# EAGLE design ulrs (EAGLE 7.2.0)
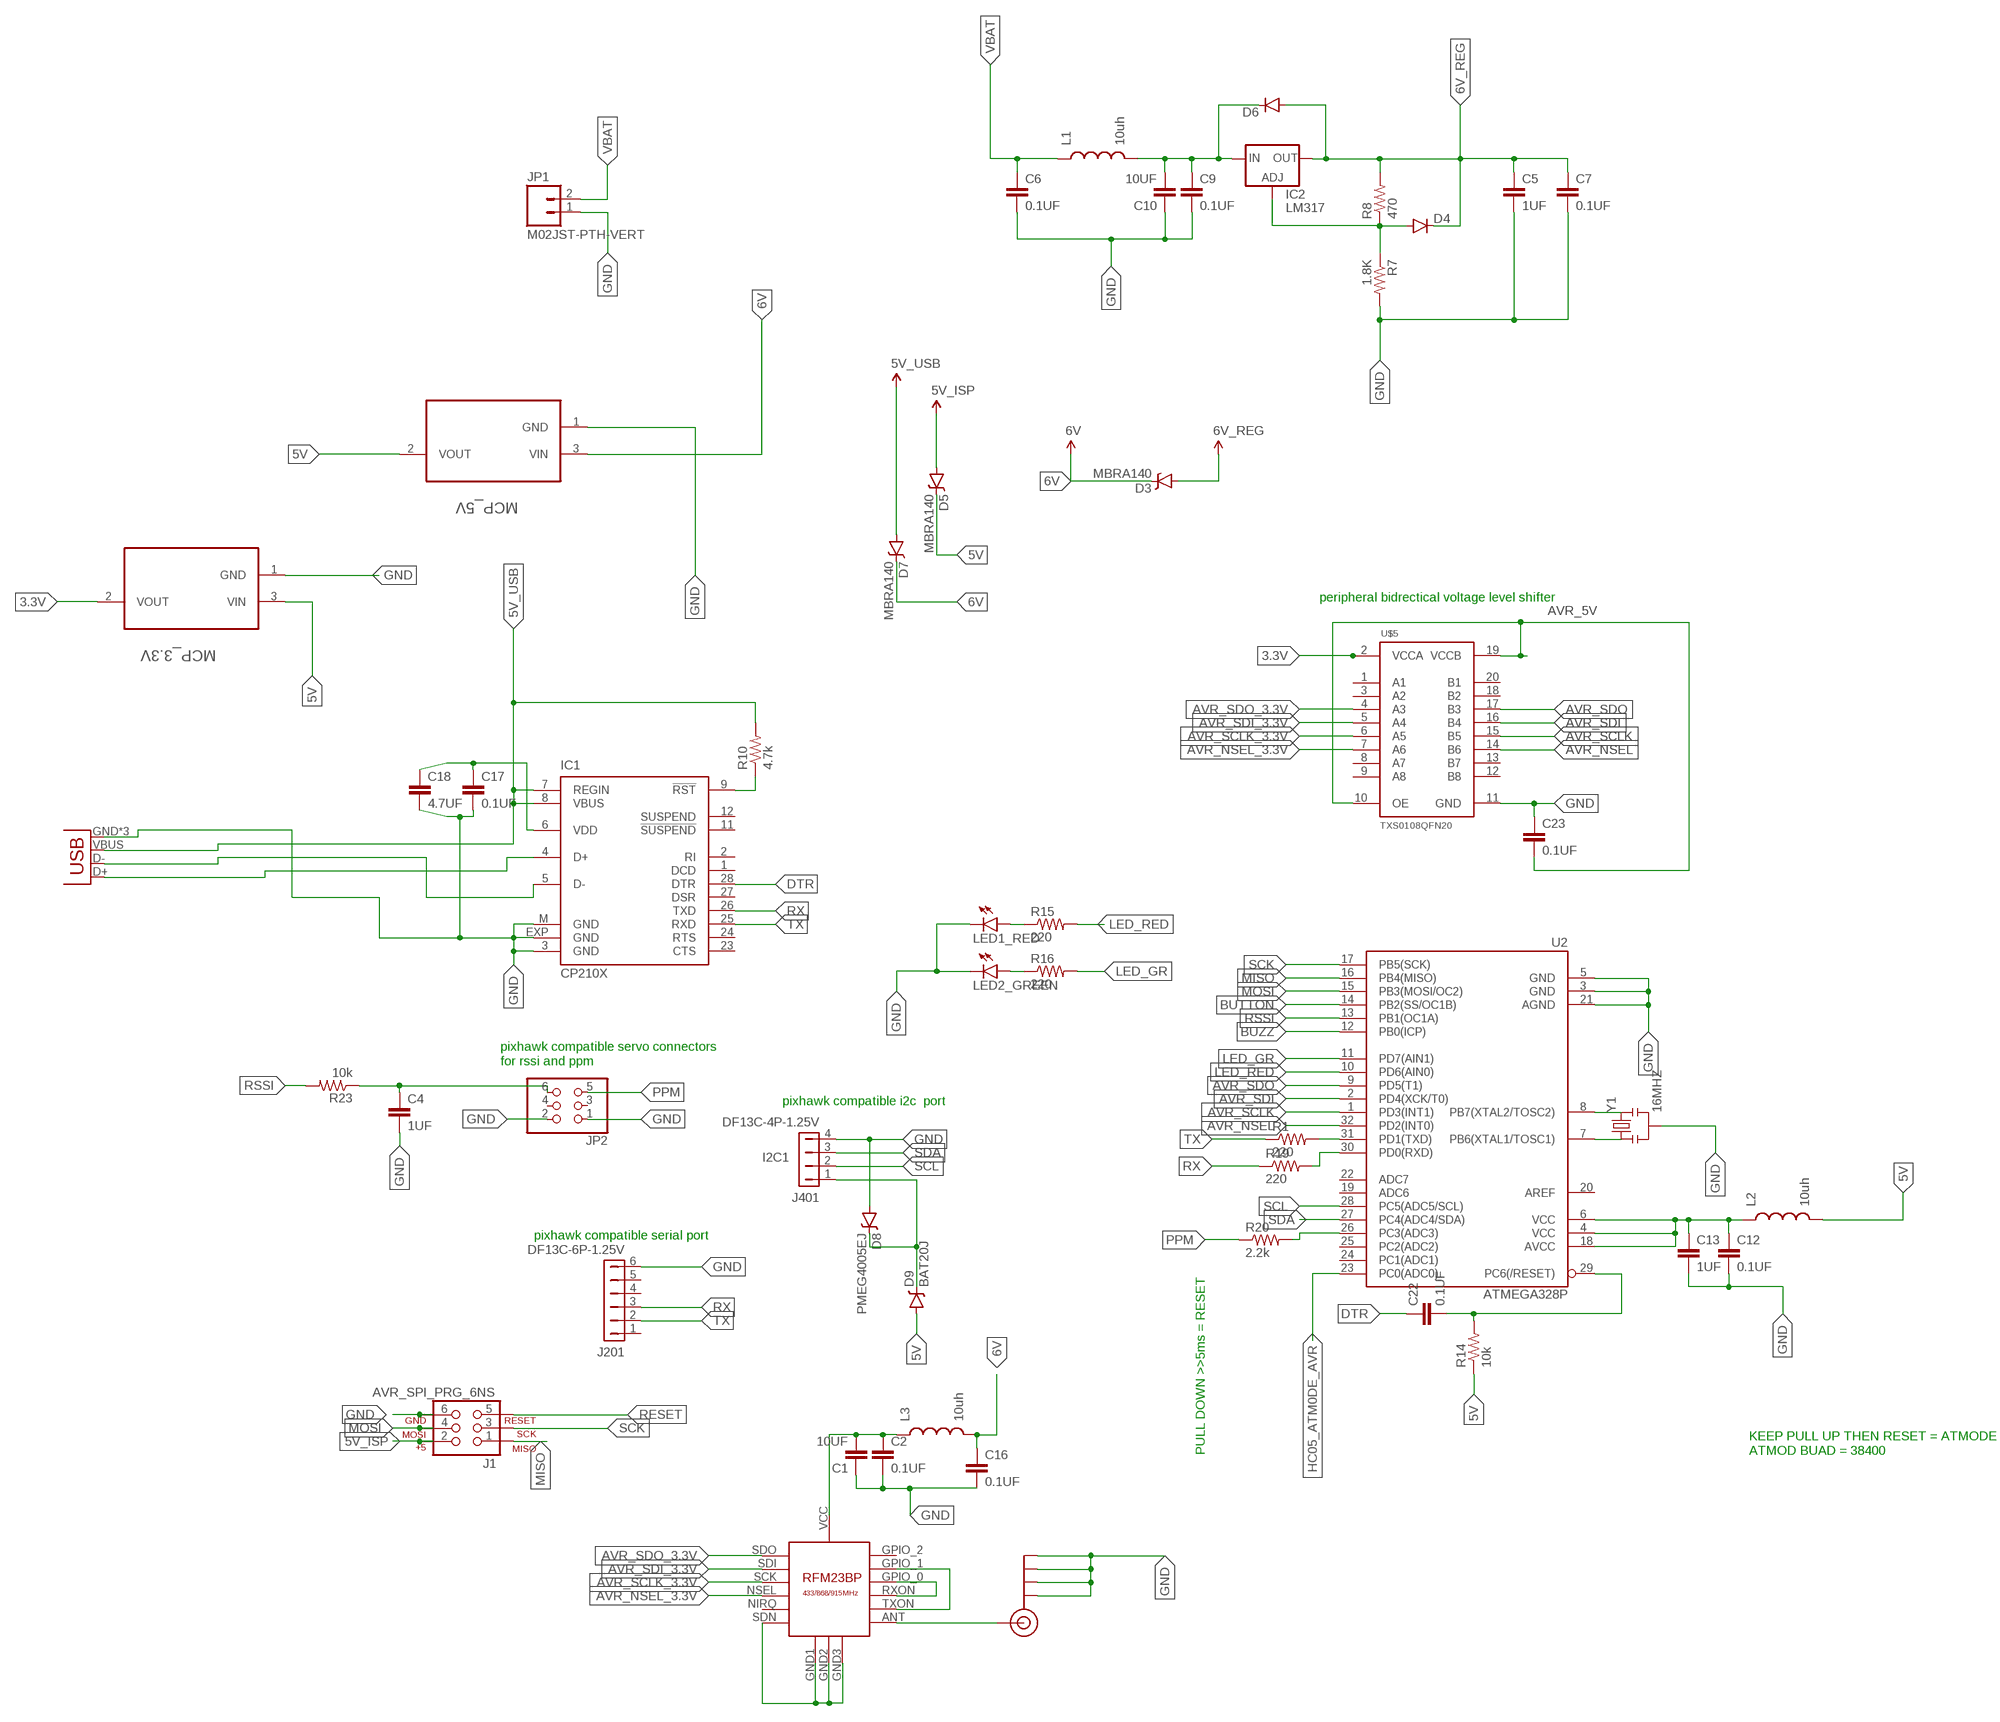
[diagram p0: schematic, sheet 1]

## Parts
C1  10UF  CAP0805  [0805]
C2  0.1UF  CAP0402-CAP  [0402-CAP]
C4  1UF  CAP0402-CAP  [0402-CAP]
C5  1UF  CAP0402-CAP  [0402-CAP]
C6  0.1UF  CAP0402-CAP  [0402-CAP]
C7  0.1UF  CAP0402-CAP  [0402-CAP]
C9  0.1UF  CAP0402-CAP  [0402-CAP]
C10  10UF  CAP1206  [1206]
C12  0.1UF  CAP0402-CAP  [0402-CAP]
C13  1UF  CAP0402-CAP  [0402-CAP]
C16  0.1UF  CAP0402-CAP  [0402-CAP]
C17  0.1UF  CAP0402-CAP  [0402-CAP]
C18  4.7UF  CAP0402-CAP  [0402-CAP]
C22  0.1UF  CAP0402-CAP  [0402-CAP]
C23  0.1UF  CAP0402-CAP  [0402-CAP]
D3  MBRA140  DIODE-SCHOTTKY-MBRA140  [SMA-DIODE]
D4  DIODESMA  [SMA-DIODE]
D5  MBRA140  DIODE-SCHOTTKY-MBRA140  [SMA-DIODE]
D6  DIODESMA  [SMA-DIODE]
D7  MBRA140  DIODE-SCHOTTKY-MBRA140  [SMA-DIODE]
D8  PMEG4005EJ  DIODE-SCHOTTKY-PMEG4005EJ  [SOD-323]
D9  BAT20J  DIODE-SCHOTTKY-BAT20J  [SOD-323]
IC1  CP210X  CP210X_USB_UART  [MLP28]
IC2  LM317  LM317MBSTT3  [SOT223]
J1  AVR_SPI_PRG_6NS  [2X3-NS]
J201  DF13C-6P-1.25V  DF13-6P-1.25V  [DF13C-6P-1.25V]
J401  DF13C-4P-1.25V  DF13-4P-1.25V  [DF13C-4P-1.25V]
J$1  SMA_EDGE  [SMA-EDGE]
JP1  M02JST-PTH-VERT  [JST-2-PTH-VERT]
JP2  PINHD-2X3  [2X03]
JP3  USB-MICROB  [USB-MICROB]
L1  10uh  INDUCTOR1007  [1007]
L2  10uh  INDUCTOR1007  [1007]
L3  10uh  INDUCTOR1007  [1007]
LED1_RED  LED0603  [LED-0603]
LED2_GREEN  LED0603  [LED-0603]
MCP_3.3V  MCP1700T-3302E/TT  [SOT95P237X112-3N]
MCP_5V  MCP1700T-5002E/TT  [SOT95P237X112-3N]
R1  220  RESISTOR0603-RES  [0603-RES]
R7  1.8K  RESISTOR0603-RES  [0603-RES]
R8  470  RESISTOR0603-RES  [0603-RES]
R10  4.7k  RESISTOR0603-RES  [0603-RES]
R14  10k  RESISTOR0603-RES  [0603-RES]
R15  220  RESISTOR0603-RES  [0603-RES]
R16  220  RESISTOR0603-RES  [0603-RES]
R19  220  RESISTOR0603  [0603-RES]
R20  2.2k  RESISTOR0603-RES  [0603-RES]
R23  10k  RESISTOR0603-RES  [0603-RES]
U2  ATMEGA328P  ATMEGA328_SMT  [TQFP32-08]
U$3  RFM23BP  [RFM23BP]
U$5  TXS0108QFN20  [QFN20-RGY]
Y1  16MHZ  RESONATOR16MHZ  [RESONATOR-SMD]

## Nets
3.3V: MCP_3.3V.2(VOUT) U$5.2(VCCA)
5V: D5.C D9.A L2.2 MCP_3.3V.3(VIN) MCP_5V.2(VOUT) R14.1
5V_ISP: D5.A J1.2
5V_USB: D7.A IC1.7(REGIN) IC1.8(VBUS) JP3.VBUS R10.2
6V: C16.1 D3.C D7.C L3.2 MCP_5V.3(VIN)
6V_REG: C5.1 C7.1 D3.A D4.C D6.A IC2.4(OUT) R8.2
AVR_5V: C12.1 C13.1 C23.2 L2.1 U2.4(VCC) U2.6(VCC) U2.18(AVCC) U$5.10(OE) U$5.19(VCCB)
AVR_NSEL: U2.32(PD2(INT0)) U$5.14(B6)
AVR_NSEL_3.3V: U$3.NSEL U$5.7(A6)
AVR_SCLK: U2.1(PD3(INT1)) U$5.15(B5)
AVR_SCLK_3.3V: U$3.SCK U$5.6(A5)
AVR_SDI: U2.2(PD4(XCK/T0)) U$5.16(B4)
AVR_SDI_3.3V: U$3.SDI U$5.5(A4)
AVR_SDO: U2.9(PD5(T1)) U$5.17(B3)
AVR_SDO_3.3V: U$3.SDO U$5.4(A3)
BUTTON: U2.14(PB2(SS/OC1B))
BUZZ: U2.12(PB0(ICP))
DTR: C22.1 IC1.28(DTR)
GND: C1.1 C2.2 C4.2 C5.2 C6.2 C7.2 C9.2 C10.1 C12.2 C13.2 C16.2 C17.2 C18.2 C23.1 D8.A IC1.3(GND) IC1.EXP(GND) IC1.M(GND) J1.6 J201.6 J401.4 J$1.GND@0(GND) J$1.GND@1(GND) J$1.GND@2(GND) J$1.GND@3(GND) JP1.1 JP2.1 JP2.2 JP3.GND JP3.MT1(GND) JP3.MT2(GND) LED1_RED.C LED2_GREEN.C MCP_3.3V.1(GND) MCP_5V.1(GND) R7.2 U2.3(GND) U2.5(GND) U2.21(AGND) U$3.GND1 U$3.GND2 U$3.GND3 U$3.SDN U$5.11(GND) Y1.2
HC05_ATM0DE_AVR: U2.23(PC0(ADC0))
LED_GR: R16.2 U2.11(PD7(AIN1))
LED_RED: R15.2 U2.10(PD6(AIN0))
MISO: J1.1 U2.16(PB4(MISO))
MOSI: J1.4 U2.15(PB3(MOSI/OC2))
N$1: C9.1 C10.2 D6.C IC2.3(IN) L1.2
N$3: D4.A IC2.1(ADJ) R7.1 R8.1
N$6: IC1.5(D-) JP3.D-
N$7: U2.8(PB7(XTAL2/TOSC2)) Y1.3
N$8: U2.7(PB6(XTAL1/TOSC1)) Y1.1
N$13: IC1.4(D+) JP3.D+
N$14: C1.2 C2.1 L3.1 U$3.VCC
N$18: U$3.GPIO_0 U$3.RXON
N$19: U$3.GPIO_1 U$3.TXON
N$21: J$1.SIG(SIGNAL) U$3.ANT
N$28: IC1.9(!RST) R10.1
N$29: C17.1 C18.1 IC1.6(VDD)
N$31: LED1_RED.A R15.1
N$34: LED2_GREEN.A R16.1
N$35: R1.2 U2.31(PD1(TXD))
N$38: R20.2 U2.26(PC3(ADC3))
N$41: D8.C D9.C J401.1
N$43: R19.2 U2.30(PD0(RXD))
N$44: C4.1 JP2.6 R23.1
PPM: JP2.5 R20.1
RESET: C22.2 J1.5 R14.2 U2.29(PC6(/RESET))
RSSI: R23.2 U2.13(PB1(OC1A))
RX: IC1.26(TXD) J201.3 R19.1
SCK: J1.3 U2.17(PB5(SCK))
SCL: J401.2 U2.28(PC5(ADC5/SCL))
SDA: J401.3 U2.27(PC4(ADC4/SDA))
TX: IC1.25(RXD) J201.2 R1.1
VBAT: C6.1 JP1.2 L1.1
Unconnected: IC1.1(DCD) IC1.2(RI) IC1.11(!SUSPEND) IC1.12(SUSPEND) IC1.23(CTS) IC1.24(RTS) IC1.27(DSR) J201.1 J201.4 J201.5 JP2.3 JP2.4 U2.19(ADC6) U2.20(AREF) U2.22(ADC7) U2.24(PC1(ADC1)) U2.25(PC2(ADC2)) U$3.GPIO_2 U$3.NIRQ U$5.1(A1) U$5.3(A2) U$5.8(A7) U$5.9(A8) U$5.12(B8) U$5.13(B7) U$5.18(B2) U$5.20(B1)

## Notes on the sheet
- peripheral bidrectical voltage level shifter
- pixhawk compatible servo connectors
  for rssi and ppm
- pixhawk compatible i2c  port
- I2C1
- pixhawk compatible serial port
- PULL DOWN >>5ms = RESET
- KEEP PULL UP THEN RESET = ATMODE
  ATMOD BUAD = 38400

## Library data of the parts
C1 C10 = SparkFun-Capacitors:CAP: Capacitor
C2 C4-C7 C9 C12 C13 C16-C18 C22 C23 = SparkFun-Passives:CAP: Capacitor
D3 D5 D7 = SparkFun-DiscreteSemi:DIODE-SCHOTTKY: Schottky diodes in SFE's production catalog; PROD_ID: DIO-08053
D4 D6 = SparkFun-DiscreteSemi:DIODE: Diode
D8 = SparkFun-DiscreteSemi:DIODE-SCHOTTKY: Schottky diodes in SFE's production catalog; PROD_ID: DIO-10955
D9 = SparkFun-DiscreteSemi:DIODE-SCHOTTKY: Schottky diodes in SFE's production catalog; PROD_ID: DIO-11623
IC1 = SparkFun-DigitalIC:CP210X_USB_UART: Single-Chip USB to UART Bridge Source: www.silabs.com .. CP2101.pdf / cp2102.pdf. Spark Fun Electronics SKU : COM-00310
IC2 = v-reg:LM317?*: 500 mA Adjustable Output Positive Voltage Regulator Source: http://www.onsemi.co.jp .. LM317M-D.PDF
J1 = SparkFun-Connectors:AVR_SPI_PRG_6: AVR ISP 6 Pin This is the reduced ISP connector for AVR programming. Common on Arduino. This footprint will take up less PCB space and can be used with a 10-pin to 6-pin adapter such as SKU: BOB-08508 **Special note about "TEST_POINT" package. The stop mask is on the top side, so if you want your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
J201 = con-hirose-df13:DF13-6P-1.25: DF13-6P 1.25mm Pitch Miniature Crimping Connector.; PARTNO: DF13C-6P-1.25V(20)
J401 = con-hirose-df13:DF13-4P-1.25: DF13-4P 1.25mm Pitch Miniature Crimping Connector.; PARTNO: DF13C-4P-1.25V(20)
J$1 = SparkFun-Connectors:SMA_EDGE: SMA Antenna Connector End launch SMA connector. The paste layer has been removed so that the connector can be hand soldered onto the board after reflow.
JP1 = SparkFun-Connectors:M02: Standard 2-pin 0.1" header. Use with
JP2 = pinhead:PINHD-2X3: PIN HEADER
JP3 = SparkFun-Connectors:USB: USB Connectors USB-B-PTH is fully proven SKU : PRT-00139/CONN-08278 USB-miniB is fully proven SKU : PRT-00587 USB-A-PCB is untested. USB-A-H is throughly reviewed, but untested. Spark Fun Electronics SKU : PRT-00437 USB-B-SMT is throughly reviewed, but untested. Needs silkscreen touching up.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; PROD_ID: CONN-09505
L1-L3 = SparkFun-Passives:INDUCTOR: Inductors
LED1_RED LED2_GREEN = SparkFun-LED:LED: LEDs
MCP_3.3V = Microchip_By_element14_Batch_1:MCP1700T-3302E/TT: Low Quiescent Current LDO; MPN: MCP1700T-3302E/TT; OC_FARNELL: 1296592; OC_NEWARK: 88H9817; PACKAGE: SOT23-3; SUPPLIER: Microchip
MCP_5V = Microchip_By_element14_Batch_1:MCP1700T-5002E/TT: Low Quiescent Current LDO; MPN: MCP1700T-5002E/TT; OC_FARNELL: 1296593; OC_NEWARK: 88H9819; PACKAGE: SOT23-3; SUPPLIER: Microchip
R1 R7 R8 R10 R14-R16 R19 R20 R23 = SparkFun-Resistors:RESISTOR: Resistor
U2 = SparkFun-DigitalIC:ATMEGA328_SMT: 32-Pin Atmega328 part Commonly used on Arduino compatible boards Available in QFP and QFN packages TQFP is IC-09069 QFN is non-stock; PROD_ID: IC-09069
U$3 = RFM23BP:RFM23BP: HopeRF RFM23BP Library by: http://projects.weber-itam.de
U$5 = pixhawk2:TXS0108
Y1 = SparkFun-FreqCtrl:RESONATOR: Resonator Small SMD resonator. Used, eg, on the Arduino Pro/ Pro Mini boards. 8MHz- XTAL-08895 16MHz- XTAL-08900; PROD_ID: XTAL-08900

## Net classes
0 signal: width 0.15 mm, drill 0.15 mm, clearance 0.152 mm
1 power: width 0.15 mm, drill 0.2 mm, clearance 0.152 mm

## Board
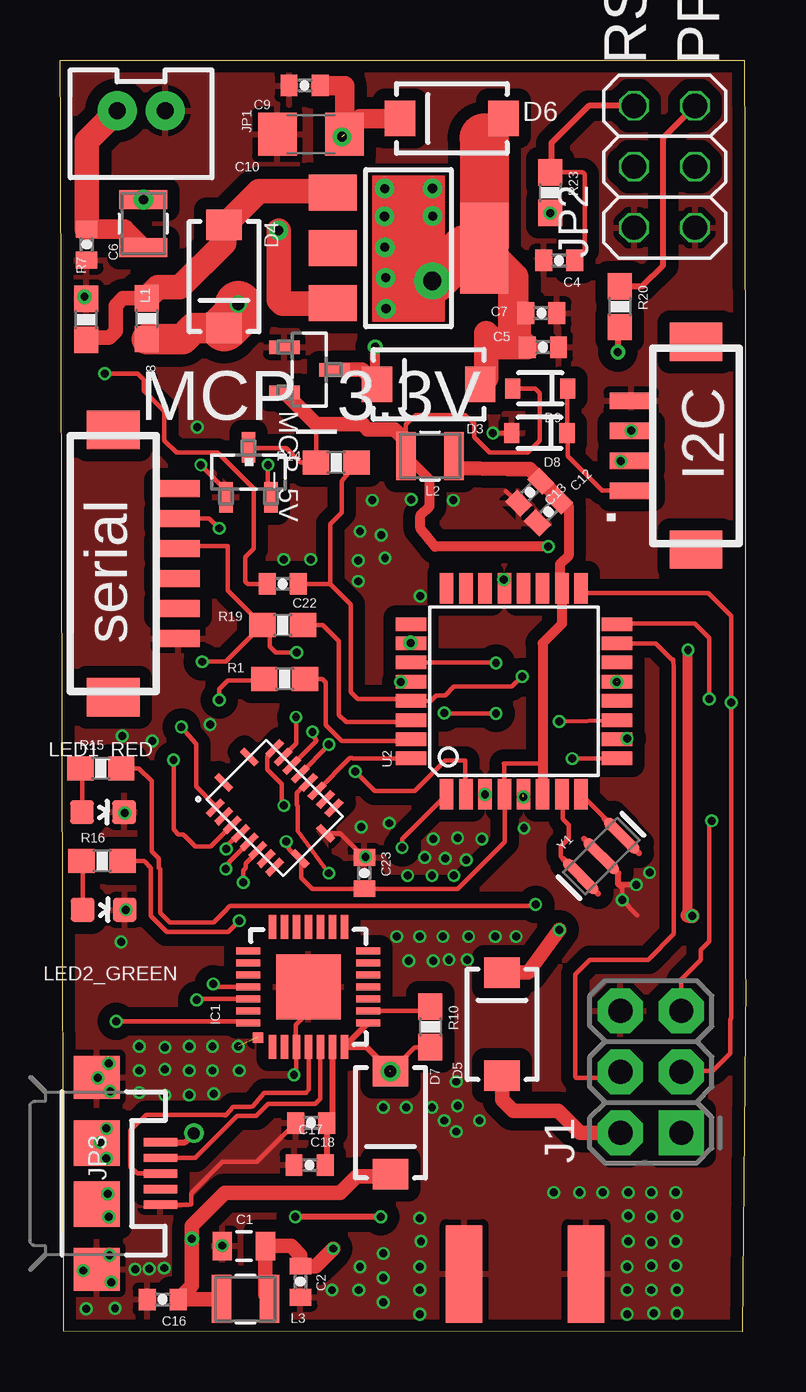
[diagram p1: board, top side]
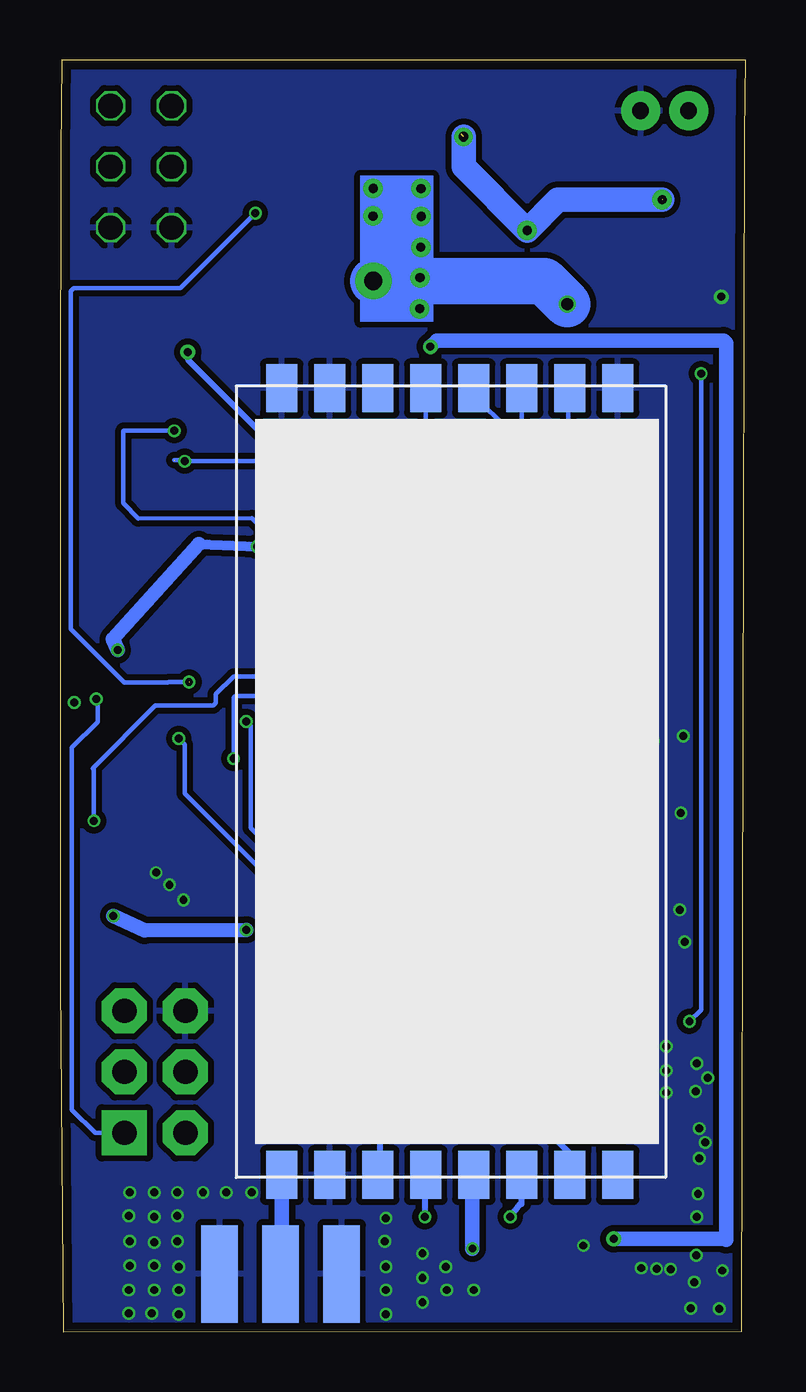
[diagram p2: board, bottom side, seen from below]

Size 28.57 x 53 mm. Coordinates in mm from the lower left corner, seen from the top.
Outline: 0.16,0.01 0.03,49.92 0,52.99 28.5,53 28.54,49.14 28.56,37.69 28.56,14.78 28.57,14.59 28.43,0 0.16,0.01
Copper layers (1*16): Top 0.0356mm / dielectric 1.5011mm / Bottom 0.0356mm
Design rules "oshpark-2layer *": minimum track width 6mil, minimum drill 13mil, track to track 6mil, track to pad 6mil, pad to pad 6mil, via to via 6mil, smd to smd 6mil, copper to edge 15mil, drill to drill 6mil, minimum pad ring 4mil, minimum via ring 4mil, stop-mask expansion 2mil, vias tented up to drill 13mil, thermal gap 10mil
tRestrict: area 21.6,18.2 to 24.2,20.9; area 20.9,18.9 to 23.6,21.6

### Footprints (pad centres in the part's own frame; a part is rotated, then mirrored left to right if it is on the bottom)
0805 = smd 0.8 x 1.2: 1 -0.9,0; 2 0.9,0
0402-CAP = smd 0.7 x 0.9: 1 -0.65,0; 2 0.65,0
1206 = smd 1.6 x 1.8: 1 -1.4,0; 2 1.4,0
SMA-DIODE = smd 1.27 x 1.47: A -2.15,0; C 2.15,0
SOD-323 = smd 0.63 x 0.83: A 1.15,0; C -1.15,0
MLP28 = smd 1 x 0.3: 1 -2.5,1.5; 2 -2.5,1; 3 -2.5,0.5; 4 -2.5,0; 5 -2.5,-0.5; 6 -2.5,-1; 7 -2.5,-1.5; 15 2.5,-1.5; 16 2.5,-1; 17 2.5,-0.5; 18 2.5,0; 19 2.5,0.5; 20 2.5,1; 21 2.5,1.5 | smd 0.3 x 1: 8 -1.5,-2.5; 9 -1,-2.5; 10 -0.5,-2.5; 11 0,-2.5; 12 0.5,-2.5; 13 1,-2.5; 14 1.5,-2.5; 22 1.5,2.5; 23 1,2.5; 24 0.5,2.5; 25 0,2.5; 26 -0.5,2.5; 27 -1,2.5; 28 -1.5,2.5 | smd 2.7 x 2.7: EXP 0,0 | smd 0.435 x 0.435: M -2.103,2.103
SOT223 = smd 1.5 x 2: 1 -2.3,-3.15; 2 0,-3.15; 3 2.3,-3.15 | smd 3.8 x 2: 4 0,3.15
2X3-NS = drill 1.016 pad 1.88 square: 1 -2.54,-1.27 | drill 1.016 pad 1.88 octagon: 2 -2.54,1.27; 3 0,-1.27; 4 0,1.27; 5 2.54,-1.27; 6 2.54,1.27
DF13C-6P-1.25V = smd 0.7 x 1.8: 1 -3.125,0.9; 2 -1.875,0.9; 3 -0.625,0.9; 4 0.625,0.9; 5 1.875,0.9; 6 3.125,0.9 | smd 1.6 x 2.2: M$0 5.575,-1.8; M$1 -5.575,-1.8
DF13C-4P-1.25V = smd 0.7 x 1.8: 1 -1.875,0.9; 2 -0.625,0.9; 3 0.625,0.9; 4 1.875,0.9 | smd 1.6 x 2.2: M$0 4.325,-1.8; M$1 -4.325,-1.8
SMA-EDGE = smd 1.524 x 4.064: GND@0 0,0; GND@1 5.08,0; SIG 2.54,0 | smd 1.524 x 4.064 bottom: GND@2 0,0; GND@3 5.08,0
JST-2-PTH-VERT = drill 0.7 pad 1.626: 1 -1,-0.55; 2 1,-0.55
2X03 = drill 1.016 octagon: 1 -2.54,-1.27; 2 -2.54,1.27; 3 0,-1.27; 4 0,1.27; 5 2.54,-1.27; 6 2.54,1.27
USB-MICROB = smd 0.35 x 1.4: D+ 0,2.65; D- -0.65,2.65; GND 1.3,2.65; ID 0.65,2.65; VBUS -1.3,2.65 | smd 1.8 x 1.9: MT1 -4,0; MT2 4,0 | smd 1.9 x 1.9: P$1 -1.27,0; P$2 1.27,0
1007 = smd 2 x 0.8: 1 0,1; 2 0,-1
LED-0603 = smd 1 x 1: A 0,-0.877; C 0,0.877
SOT95P237X112-3N = smd 0.559 x 1.27: 1 -0.94,-1.041; 2 0.94,-1.041; 3 0,1.041
0603-RES = smd 1.1 x 1: 1 -0.85,0; 2 0.85,0
TQFP32-08 = smd 1.27 x 0.559: 1 -4.293,2.8; 2 -4.293,2; 3 -4.293,1.2; 4 -4.293,0.4; 5 -4.293,-0.4; 6 -4.293,-1.2; 7 -4.293,-2; 8 -4.293,-2.8; 17 4.293,-2.8; 18 4.293,-2; 19 4.293,-1.2; 20 4.293,-0.4; 21 4.293,0.4; 22 4.293,1.2; 23 4.293,2; 24 4.293,2.8 | smd 0.559 x 1.27: 9 -2.8,-4.293; 10 -2,-4.293; 11 -1.2,-4.293; 12 -0.4,-4.293; 13 0.4,-4.293; 14 1.2,-4.293; 15 2,-4.293; 16 2.8,-4.293; 25 2.8,4.293; 26 2,4.293; 27 1.2,4.293; 28 0.4,4.293; 29 -0.4,4.293; 30 -1.2,4.293; 31 -2,4.293; 32 -2.8,4.293
RFM23BP = smd 2 x 1.3: ANT 16.9,-7.5; GND1 -15.9,6.5; GND2 -15.9,-7.5; GND3 16.9,-5.5; GPIO_0 16.9,2.5; GPIO_1 16.9,4.5; GPIO_2 16.9,6.5; NIRQ -15.9,-3.5; NSEL -15.9,-1.5; RXON 16.9,-1.5; SCK -15.9,0.5; SDI -15.9,2.5; SDN -15.9,-5.5; SDO -15.9,4.5; TXON 16.9,-3.5; VCC 16.9,0.5
QFN20-RGY = smd 0.28 x 0.85: 1 -0.75,2.25; 10 -0.75,-2.25; 11 0.75,-2.25; 20 0.75,2.25 | smd 0.85 x 0.28: 2 -1.75,1.75; 3 -1.75,1.25; 4 -1.75,0.75; 5 -1.75,0.25; 6 -1.75,-0.25; 7 -1.75,-0.75; 8 -1.75,-1.25; 9 -1.75,-1.75; 12 1.75,-1.75; 13 1.75,-1.25; 14 1.75,-0.75; 15 1.75,-0.25; 16 1.75,0.25; 17 1.75,0.75; 18 1.75,1.25; 19 1.75,1.75
RESONATOR-SMD = smd 0.45 x 1.905: 1 -1.2,0; 2 0,0; 3 1.2,0

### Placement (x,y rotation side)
C1  7.66,3.57 0 top
C2  10.02,2.08 270 top
C4  20.8,44.64 180 top
C5  20.12,41.03 0 top
C6  1.11,45.3 270 top
C7  20.05,42.45 0 top
C9  10.19,51.94 180 top
C10  10.46,49.9 0 top
C12  20.35,34.17 225 top
C13  19.57,34.99 225 top
C16  4.28,1.34 180 top
C17  10.4,6.94 180 top
C18  10.47,8.69 180 top
C22  9.28,31.17 0 top
C23  12.68,19.11 270 top
D3  15.36,39.48 180 top
D4  6.84,43.98 270 top
D5  18.42,12.81 90 top
D6  16.33,50.56 180 top
D7  13.77,8.71 270 top
D8  19.98,37.45 180 top
D9  20.01,39.31 180 top
IC1  10.35,14.36 90 top
IC2  14.52,45.16 270 top
J1  24.62,10.82 90 top
J201  4.02,32.01 270 top
J401  24.7,36.92 90 top
J$1  21.92,2.4 0 bottom
JP1  3.38,50.34 180 top
JP2  25.19,48.55 90 top
JP3  1.53,6.59 270 top
L1  3.47,46.18 180 top
L2  15.42,36.49 270 top
L3  7.73,1.36 270 top
LED1_RED  1.8,21.65 270 top
LED2_GREEN  1.82,17.58 270 top
MCP_3.3V  7.85,35.82 0 top
MCP_5V  10.39,40.09 270 top
R1  9.36,27.2 0 top
R7  1.09,42.18 90 top
R8  3.62,42.21 270 top
R10  15.44,12.7 270 top
R14  11.51,36.22 0 top
R15  1.7,23.48 0 top
R16  1.75,19.61 0 top
R19  9.28,29.44 0 top
R20  23.33,42.72 270 top
R23  20.43,47.47 270 top
U2  18.91,26.69 90 top
U$3  11.83,23.42 270 bottom
U$5  8.94,21.83 45 top
Y1  22.55,19.81 45 top

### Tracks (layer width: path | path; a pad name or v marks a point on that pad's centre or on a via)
3.3V  (via drill 0.33)
  Top 0.178: U$5.2 6.47,21.91 5.67,22.71 5.67,24.49 v5.06,25.2 | v8.67,36.12 8.67,34.9 MCP_3.3V.2
  Bottom 0.178: v5.06,25.2 5.06,28.15 5.72,28.86 5.72,32.92 5.06,33.58 5.06,34.04 5.72,34.7 7.14,34.7 8.31,35.87 8.41,35.87 v8.67,36.12
5V  (via drill 0.33 pad 0.25)
  Top 0.178: 10.65,37.82 10.68,37.82 10.68,36.24 R14.1 10.04,36.22 9.43,36.83 7.88,36.83 MCP_3.3V.3 | D9.A 19.8,39.31 19.99,39.12 19.99,37.14 19.49,36.63 17.91,36.63 17.25,37.29 17.25,37.85 16.9,38.2 14.81,38.2 14.41,37.8 14.41,37.14 14.41,36.5 L2.2
  Top 0.406: 26.17,17.35 v26.17,28.4 | v20.35,32.72 15.63,32.72 15.02,33.48 15.02,34.01 15.4,34.39 15.4,35.51 L2.2
  Top 0.61: 9.29,39.09 MCP_5V.2 10.68,37.82 12.61,37.82 12.83,37.59 13.95,37.59 14.41,37.14 | D5.C 19.51,14.96 v20.81,16.74 | v26.34,17.33 26.27,17.33 26.17,17.35
  Bottom 0.406: 22.79,32.82 v20.35,32.72
  Bottom 0.61: v20.81,16.74 25.05,16.72 v26.34,17.33 | v26.17,28.4 26.37,28.86 22.79,32.82
5V_ISP
  Top 0.61: D5.A 18.42,9.65 18.88,9.2 20.76,9.2 21.67,8.28 J1.2
5V_USB  (via drill 0.5 pad 0.81)  (1 unrouted)
  Top 0.178: R10.2 14.78,11.85 v13.77,10.84
  Top 0.254: JP3.VBUS 5.21,7.89 v5.58,8.26 | D7.A 12.76,11.86 IC1.7 IC1.8
  Bottom 0.61: v5.58,8.26 6.48,8.26 7.6,9.38 12.31,9.38 v13.77,10.84
6V  (via drill 0.33 pad 0.61)
  Top 0.406: 13.09,39.6 13.14,39.66 v13.14,41.05
  Top 0.61: L3.2 6.73,1.34 C16.1 5.5,1.9 v5.5,3.86 5.5,3.89 5.5,4.42 6.86,5.78 11.68,5.78 12.37,6.48 13.69,6.48 D7.C | MCP_5V.3 12.6,40.09 13.09,39.6 D3.C
  Bottom 0.61: v13.14,41.05 12.88,41.3 0.92,41.3 0.82,41.2 0.82,3.81 0.87,3.86 v5.5,3.86
6V_REG  (via drill 0.5, 0.76 pad 1.52)
  Top 0.254: C7.1 19.11,41.91 18.88,41.91
  Top 1.016: 19.11,41.91 19.11,41.39 C5.1 18.34,41.03 17.76,41.61 17.76,39.73 D3.A
  Top 1.27: D6.A 17.67,49.75 | IC2.4 18.88,43.95 18.88,41.91 | R8.2 5.11,41.37 5.56,41.83 D4.C
  Top 1.93: D4.C 7.43,42.41 v7.43,42.82 | v15.51,43.79 16.88,45.16 IC2.4
  Top 2.032: 17.67,49.75 IC2.4
  Bottom 1.93: v7.43,42.82 8.4,43.79 v15.51,43.79
AVR_5V  (via drill 0.33 pad 0.25)
  Top 0.178: U$5.19 8.63,23.99 8.63,23.42 9.23,22.82 9.23,22.02 v9.33,21.92 | v9.43,20.42 9.53,20.32 9.53,20.12 9.94,19.7 U$5.10 10.05,19.66 10.05,18.91 10.5,18.46 C23.2 16.58,18.46 18.52,20.4 18.52,22.39 U2.4 18.51,23.66 18.5,23.68 20.09,23.68 20.11,23.7
  Top 0.406: U2.6 20.11,23.7 20.11,28.7 20.91,29.49 U2.18 20.83,31.06 20.83,31.98 21.19,32.34 21.19,34.42 20.51,35.1 20.43,35.1
  Top 0.61: 19.58,35.95 20.43,35.1 C12.1 | 19.58,35.95 18.69,35.96 16.44,35.98 L2.1 | C13.1 19.58,35.95
  Bottom 0.178: v9.43,20.42 9.33,20.52 v9.33,21.92
AVR_NSEL
  Top 0.178: U$5.14 12.08,23.9 12.17,23.9 12.19,23.89 U2.32
AVR_NSEL_3.3V  (via drill 0.33 pad 0.25)
  Top 0.178: v7.63,18.72 7.63,19.22 7.73,19.32 7.73,19.52 8.24,20.03 U$5.7
  Bottom 0.178: v7.63,18.72 8.13,19.12 8.13,20.12 8.63,20.62 8.63,32.22 10.43,34.02 10.43,37.12 10.63,37.32 12.83,37.32 13.33,37.82 U$3.NSEL
AVR_SCLK  (via drill 0.33)
  Top 0.178: U$5.15 10.29,22.89 9.86,22.46 9.86,21.95 9.91,21.9 9.91,20.86 v11.21,19.1 | v14.25,20.17 14.25,20.54 U2.1
  Bottom 0.178: v11.21,19.1 13.64,19.1 v14.25,20.17
AVR_SCLK_3.3V  (via drill 0.33 pad 0.25)
  Top 0.178: v6.91,19.28 7.07,19.59 U$5.6
  Bottom 0.178: U$3.SCK 11.33,39.02 9.86,37.54 9.86,34.29 8.06,32.49 8.06,20.55 7.09,19.59 7.09,19.36 v6.91,19.28
AVR_SDI  (via drill 0.33 pad 0.25)
  Top 0.178: U2.2 16.9,22.41 16.9,23.8 16.06,23.8 14.79,22.53 13.11,22.53 v12.3,23.34 | v11.21,24.46 11.21,24.44 U$5.16
  Bottom 0.178: v12.3,23.34 12.3,23.37 v11.21,24.46
AVR_SDI_3.3V  (via drill 0.33 pad 0.25)
  Top 0.178: U$5.5 7.63,20.87 7.63,20.92 6.93,20.22 v6.93,20.12
  Bottom 0.178: v6.93,20.12 7.53,21.22 7.53,32.72 9.33,34.52 U$3.SDI
AVR_SDO  (via drill 0.33 pad 0.25)
  Top 0.178: U2.9 v21.35,23.89 v21.34,23.88 | v18.17,25.76 16.03,25.76 v16.01,25.78 | v10.52,25 10.67,24.62 U$5.17
  Bottom 0.178: v21.34,23.88 21.34,26.42 21.26,26.49 18.9,26.49 v18.17,25.76 | v16.01,25.78 11.26,25.73 v10.52,25
AVR_SDO_3.3V  (via drill 0.33 pad 0.25)
  Top 0.178: U$5.4 6.28,20.22 5.63,20.22 5.13,20.72 4.93,20.72 4.73,20.92 v4.73,23.82
  Bottom 0.178: v4.73,23.82 4.53,23.92 4.63,34.25 4.73,34.34 4.73,34.37 5.47,35.11 6.86,35.11 7.4,35.64 7.4,39.26 U$3.SDO
DTR  (via drill 0.33 pad 0.25)
  Top 0.178: C22.1 7.83,31.16 7.73,31.27 7.73,32.29 8.08,32.64 8.08,35.13 6.58,36.63 4.86,36.63 4.35,37.14 4.35,38.36 3.48,39.22 3.48,39.68 3.23,39.93 v1.86,39.93 | v2.34,12.93 7.78,12.93 IC1.28
  Bottom 0.178: v1.86,39.93 1.86,13.41 v2.34,12.93
GND  (via drill 0.33, 0.33 pad 0.25, 0.33 pad 0.61)  (3 unrouted)
  Top 0.178: C13.2 18.57,35.03 18.59,35.01 | v9.75,10.7 9.85,10.8 IC1.3 9.82,11.89 9.82,12.77 10.35,13.3 IC1.EXP | U$5.11 11.67,20.77 C23.1 | U2.21 18.51,31.33 v18.5,31.35 | D8.A 18.81,37.44 v18.04,37.44 | C18.2 8.19,7.06 6.76,7.06 5.47,5.77 5.47,5.31 5.36,5.29 JP3.GND | MCP_3.3V.1 6.91,35.08 v5.87,36.12 | 24.06,17.35 v23.42,17.99 23.42,18.47 23.27,18.62
  Top 0.254: v24.01,18.62 23.27,18.62 23.27,19.1
  other vias: 1.02,43.13 12.73,19.79 19.31,22.28 17.71,22.38 2.54,16.23 2.75,17.58 2.7,21.62 3.84,24.62 2.6,24.82 6.25,25.3 4.35,2.64 3.13,2.59 3.71,2.62 1.99,5.74 2.04,4.78 1.94,8.46 1.94,7.22 1.68,7.88 1.1,0.94 2.29,0.97 2.06,3.18 2.14,2.06 0.97,2.54 6.76,3.58 13.39,33.2 12.5,33.35 16.39,34.65 14.63,34.67 13.01,34.65 5.72,37.7 19.33,20.98 24.57,19.13 23.63,0.71 23.63,1.73 23.63,2.7 23.68,3.76 23.68,4.83 23.68,5.79 22.61,5.79 21.65,5.79 20.58,5.79 14.99,0.71 14.99,1.73 14.99,2.7 15.04,3.76 14.99,4.73 13.47,3.25 13.47,2.24 13.47,1.22 12.5,2.7 12.45,1.73 11.33,1.73 24.74,0.76 24.64,1.73 24.64,2.75 24.64,3.71 24.64,4.78 24.64,5.79 25.66,5.79 25.71,4.83 19,16.46 18.14,16.46 17.02,16.46 15.96,16.46 14.99,16.46 14.03,16.46 14.53,15.45 15.55,15.45 16.21,15.5 16.97,15.5 16.51,10.42 16.57,9.4 17.48,8.79 16.01,8.79 16.51,8.33 15.5,9.35 14.43,9.35 13.47,9.35 25.66,3.76 25.66,2.75 25.71,1.73 25.71,0.76 7.42,11.89 7.47,10.87 6.41,9.91 6.35,10.87 6.35,11.89 5.39,11.89 5.39,10.87 5.39,9.86 4.37,9.86 4.37,10.92 4.37,11.84 3.31,11.89 3.31,10.87 3.31,9.96 17.58,20.53 16.57,20.58 15.55,20.53 13.72,21.19 14.48,19 15.5,19 16.41,19 16.92,19.66 16.06,19.71 15.19,19.76 12.55,21.03 15.02,30.66 12.43,32.13 13.54,32.24 12.43,31.27 10.44,32.18 9.33,32.18 2.04,11.18 1.58,10.57 2.09,10.01
  pour Top (isolate 0.508): 28.22,52.72 0.21,52.72 0.21,52.56 0.35,52.56 0.35,0.83 0.28,0.83 0.28,0.16 28.26,0.16 28.26,0.18 28.31,0.18 28.31,52.34 28.27,52.34 28.27,52.72 28.26,52.72 28.26,52.73
  pour Bottom: 28.36,52.83 28.36,52.84 28.29,52.84
  pour Bottom (isolate 0.254): 28.05,0.26 0.33,0.26 0.33,0.28 0.26,0.28 0.26,52.71 28.27,52.71 28.27,52.05 28.22,52.05 28.22,0.49 28.22,0.38 28.1,0.26
LED_GR  (via drill 0.33 pad 0.25)
  Top 0.178: R16.2 3.51,19.61 3.79,19.33 3.79,17.33 4.45,16.66 7.02,16.66 v7.47,17.12 | v20.81,25.43 23.2,25.48 U2.11
  Bottom 0.178: v7.47,17.12 16.87,17.12 18.6,18.85 18.6,18.95 20.63,20.98 20.63,25.25 v20.81,25.43
LED_RED  (via drill 0.33 pad 0.25)
  Top 0.178: R15.2 3.28,23.48 3.81,22.94 3.81,20.02 4.12,19.71 4.12,19.33 4.17,19.28 4.17,17.45 4.58,17.05 6.41,17.05 6.96,17.6 6.96,17.63 7.07,17.73 19.74,17.73 v19.82,17.81 | U2.10 23.6,24.69 v23.63,24.72
  Bottom 0.178: v19.82,17.81 19.82,18.88 23.37,22.43 23.37,24.46 v23.63,24.72
MISO  (via drill 0.33)
  Top 0.178: U2.16 23.21,29.52 26.45,29.52 27.06,28.91 v27.06,26.37
  Bottom 0.178: J1.1 27.11,8.28 28.07,9.25 28.07,24.34 27.01,25.4 27.01,26.32 v27.06,26.37
MOSI
  Top 0.178: U2.15 24.82,28.68 25.48,28.02 25.56,28.02 25.58,27.64 25.58,16.56 24.52,15.5 22.08,15.5 21.47,14.89 21.47,10.62 21.52,10.57 23.09,10.57 J1.4
N$1  (via drill 0.38 pad 0.81, 0.41 pad 0.76)  (2 unrouted)
  Top 0.813: C9.1 11.86,51.94 C10.2 12.52,50.56 D6.C
  Top 1.016: IC2.3 9.25,42.85 9.11,42.99 v9.11,45.9
  Bottom 1.016: v11.75,49.8 11.75,48.54 v9.11,45.9 7.83,47.18 v3.48,47.18
N$3
  Top 0.406: IC2.1 11.21,47.3 11.06,47.3
  Top 0.61: R8.1 2.62,43.06 2.32,42.76 2.32,41.7 2.06,41.43 1.19,41.43 R7.1
  Top 1.016: 11.06,47.3 10.83,47.52 8.28,47.52 6.88,46.12 D4.A 6.84,45.37 5,43.52 4.08,43.52 R8.1
N$4  (via drill 0.38 pad 0.81)
  Top 0.254: v13.58,42.63 13.57,42.64 v13.57,43.92 13.54,43.96 v13.54,45.19 13.52,45.21 v13.52,46.48 v13.53,46.49 v13.53,47.64 v13.54,47.65 v15.52,47.65 15.53,47.64 v15.53,46.5
N$6
  Top 0.178: JP3.D- 5.63,7.24 7.38,8.99 8.18,8.99 8.68,9.49 10.63,9.49 10.84,9.7 IC1.5
N$7
  Top 0.178: 22.68,21.38 22.89,21.22 U2.8
N$8
  Top 0.178: U2.7 20.95,22.36 20.95,21.36 21.19,21.12 21.19,20.55 20.86,20.22 20.86,19.81 20.98,19.68
N$13
  Top 0.178: JP3.D+ 3.21,6.59 2.94,6.86 2.94,8.38 3.59,9.04 6.83,9.04 6.86,9.01 6.91,9.01 7.21,9.36 7.94,9.36 8.01,9.38 8.04,9.38 8.52,9.94 10.26,9.94 10.36,10.08 IC1.4
N$14  (via drill 0.33 pad 0.25)
  Top 0.61: L3.1 8.56,1.52 C1.2 9.64,3.57 10.01,3.19 C2.1 10.65,2.73 v11.38,3.46
  Bottom 0.61: U$3.VCC 11.38,6.47 v11.38,3.46
N$18  (via drill 0.33 pad 0.25)
  Top 0.254: v13.37,4.78 v9.81,4.78
  Bottom 0.254: U$3.RXON | U$3.GPIO_0 9.33,5.32 9.4,5.32 v9.81,4.78 | 13.37,6.48 v13.37,4.78
  Bottom 0.406: U$3.RXON 13.37,6.48
N$19
  Bottom 0.254: U$3.TXON 15.23,6.63 15.23,8.22 15.13,8.32 8.23,8.32 7.33,7.42 U$3.GPIO_1
N$21
  Bottom 0.61: U$3.ANT 19.33,2.45 J$1.SIG
N$28
  Top 0.178: IC1.9 15.17,13.36 R10.1
N$29
  Top 0.254: IC1.6 11.35,8.93 C18.1 11.12,7 C17.1
N$31
  Top 0.178: LED1_RED.A 0.92,23.41 R15.1
N$34
  Top 0.178: LED2_GREEN.A 0.94,19.57 R16.1
N$35
  Top 0.178: U2.31 14.55,24.62 11.74,24.62 11.08,25.28 11.08,27.05 10.93,27.2 R1.2
N$38  (via drill 0.33 pad 0.61)  (1 unrouted)
  Top 0.254: R20.2 23.33,41.77 23.25,41.68 v23.25,40.82
  Bottom 0.254: v23.25,40.82 23.25,40.52 13.01,30.28 13.01,28.65 13.06,28.6 13.52,28.6 13.62,28.7 v14.61,28.7
N$41
  Top 0.178: J401.1 22.6,35.05 21.16,36.49 21.16,37.43 D8.C 21.13,39.28 D9.C
N$43
  Top 0.178: U2.30 14.54,25.4 11.92,25.4 11.61,25.71 11.61,28.78 10.95,29.44 R19.2
N$44
  Top 0.178: C4.1 21.87,45.06 21.87,48.24 21.79,48.32 R23.1
  Top 0.254: JP2.6 22.03,51.09 20.48,49.53 20.48,48.37 R23.1
PPM
  Top 0.254: R20.1 24.26,43.57 25.12,44.43 25.12,49.76 JP2.5
RESET  (via drill 0.33, 0.33 pad 0.25)
  Top 0.178: 11.26,31.16 12.12,30.3 12.12,26.65 12.4,26.37 14.54,26.37 U2.29 15.44,26.29 15.68,26.52 16.06,26.52 16.41,26.88 18.83,26.88 v19.26,27.31 | 11.26,31.16 C22.2 | 11.26,31.16 11.26,33.66 11.74,34.14 11.74,35.45 R14.2 | J1.5 25.89,14.68 26.7,15.5 26.7,15.9 27.06,16.26 27.06,21.09 v27.16,21.29
  Bottom 0.178: v19.26,27.31 21.34,27.31 22.08,26.57 22.08,26.19 22.18,26.09 24.59,26.09 27.21,23.47 27.16,23.42 v27.16,21.29
RSSI  (via drill 0.33 pad 0.25)  (2 unrouted)
  Bottom 0.178: v20.43,46.61 23.55,43.49 28,43.49 28.12,43.36 28.12,29.29 25.89,27.05 24.06,27.05 24.03,27.08 v23.2,27.08
RX  (via drill 0.33 pad 0.25)
  Top 0.178: R19.1 6.99,30.88 6.99,32.74 5.03,32.74 J201.3 | 9.3,23.98 9.83,24.51 v9.83,25.61 | v9.86,28.3 9,28.3 8.74,28.55 8.74,29.13 R19.1 | IC1.26 5.73,13.86 v5.69,13.82 | v5.92,27.92 6.91,27.92 R19.1
  Bottom 0.178: v9.83,25.61 9.83,28.27 v9.86,28.3 | v5.69,13.82 5.69,18.8 5.03,19.46 5.03,23.09 5.57,23.62 5.57,27.56 v5.92,27.92
SCK  (via drill 0.33)
  Top 0.178: U2.17 21.91,30.79 27.01,30.79 27.97,29.82 v27.97,26.22 27.97,13.06 27.92,13.01 27.92,11.58 27.21,10.87 25.94,10.87 J1.3
  Bottom 0.178: J1.3 26.04,10.82
SCL  (via drill 0.33 pad 0.25)  (1 unrouted)
  Top 0.178: U2.28 14.21,27.09 v14.2,27.08
  Bottom 0.178: 23.8,36.33 23.42,36.33 v23.37,36.27 19.94,36.27 15.93,32.26 15.93,27.18 15.9,27.16 14.28,27.16 v14.2,27.08
SDA  (via drill 0.33 pad 0.25)  (1 unrouted)
  Top 0.178: U2.27 18.14,27.89 v18.17,27.87
  Bottom 0.178: v18.17,27.87 19.49,29.37 19.54,32.87 20.58,33.91 25.3,33.89 25.94,34.52 25.94,37.52 25.91,37.54 J401.3
  other vias: 23.8,37.54
TX  (via drill 0.33)
  Top 0.178: IC1.25 6.5,14.36 v6.38,14.48 | v6.63,26.32 6.63,26.77 6.99,27.13 8.44,27.13 R1.1 | J201.2 6.23,33.89 v6.63,33.48
  Bottom 0.178: v6.38,14.48 6.38,18.8 5.47,19.71 5.47,22.2 6.53,23.27 6.53,24.74 6.74,24.95 6.79,24.95 6.89,25.05 6.89,26.06 v6.63,26.32 v6.63,33.48
VBAT
  Top 0.813: L1.1 2.69,45.95 C6.1
  Top 1.016: JP1.2 1.11,49.62 C6.1
(copper drawn outside any net)
  shapes: Bottom area x1, Top area x1

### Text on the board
tNames: RSSI | PPM | I2C | serial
